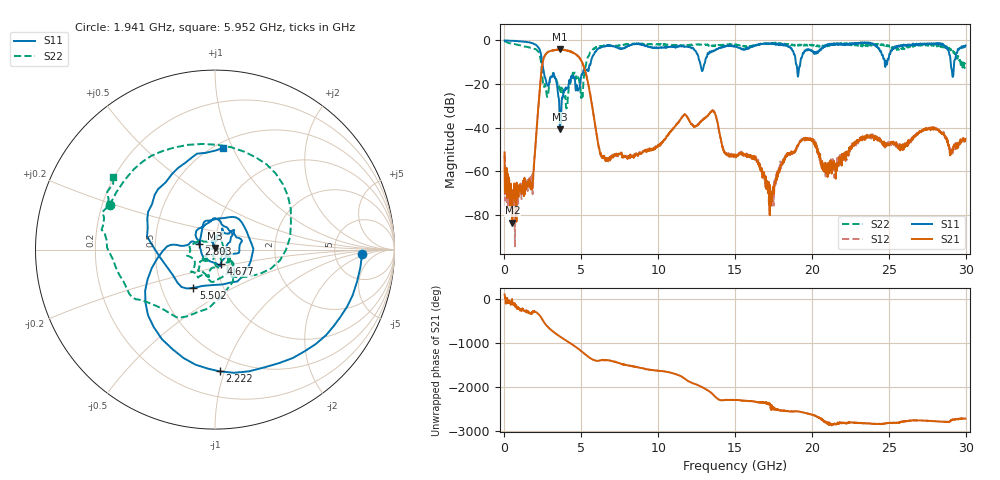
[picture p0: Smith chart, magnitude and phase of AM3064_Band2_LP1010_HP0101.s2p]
# Hz S DB R 50.0
!freq dBS11 angS11 dBS21 angS21 dBS12 angS12 dBS22 angS22
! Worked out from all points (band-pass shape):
!   1600 points, 10 MHz to 29.98 GHz, reference 50 ohm
!   highest |S21| = -4.16 dB at 3.59 GHz (marker M1); lowest = -83.5 dB at 516.1 MHz (marker M2)
!   |S21| within 3 dB of the highest: 2.613 GHz to 4.765 GHz (2.152 GHz wide, 58.3 % of centre)
!   lowest |S11| = -40.8 dB at 3.609 GHz (marker M3), VSWR 1.02, Z = 50.1 + j0.907 ohm
!   |S11| at or under -10 dB: 2.451 GHz to 5.62 GHz (3.169 GHz wide, 78.5 % of centre); 12.72 GHz to 13.05 GHz (328.9 MHz wide, 2.55 % of centre); 18.95 GHz to 19.25 GHz (303.8 MHz wide, 1.59 % of centre)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
!   |S22| runs from -31.2 to -0.3 dB; largest |S21 - S12| = 0.02
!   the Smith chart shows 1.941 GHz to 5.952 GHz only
!   S11 on the Smith chart (normalised r, x): 1.941 GHz: 10, -1; 2.222 GHz: 0.38, -0.96; 2.803 GHz: 0.83, +0.05; 4.677 GHz: 1.05, -0.17; 5.502 GHz: 0.72, -0.33; 5.952 GHz: 0.55, +0.92
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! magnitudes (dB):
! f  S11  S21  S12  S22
! 10 MHz  0.0  -51.3  -52.5  -0.3
! 516.1 MHz  -0.2  -83.5  -68.7  -1.5
! 1.941 GHz  -1.7  -55.5  -55.0  -3.9
! 2.222 GHz  -3.4  -28.9  -28.8  -5.3
! 2.803 GHz  -20.4  -5.5  -5.4  -25.7
! 3.59 GHz  -36.4  -4.2  -4.3  -22.4
! 3.609 GHz  -40.8  -4.4  -4.1  -22.8
! 4.677 GHz  -21.5  -6.6  -6.5  -16.3
! 5.015 GHz  -15.7  -9.6  -9.6  -24.5
! 5.502 GHz  -12.2  -21.9  -21.9  -6.9
! 5.952 GHz  -4.9  -41.2  -41.3  -3.2
! 6.664 GHz  -2.3  -54.1  -54.8  -2.3
! 10 GHz  -3.4  -47.9  -48.3  -1.8
! 13.54 GHz  -5.2  -32.4  -32.1  -2.6
! 15 GHz  -2.6  -52.6  -53.7  -1.8
! 16.34 GHz  -2.3  -53.2  -54.7  -2.4
! 17.35 GHz  -1.3  -74.9  -68.5  -1.2
! 18.34 GHz  -2.4  -52.6  -52.7  -1.6
! 19.99 GHz  -4.5  -46.1  -45.9  -2.0
! 20.97 GHz  -2.6  -57.2  -60.4  -2.4
! 25 GHz  -8.1  -47.8  -48.1  -2.3
! 29.98 GHz  -2.4  -45.2  -46.3  -10.2
